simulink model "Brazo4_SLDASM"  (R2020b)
settings: Solver=VariableStepAuto  StartTime=0.0  StopTime=20  RelTol=1e-3
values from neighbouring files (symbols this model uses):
  q = [q 0]    [robotSimulation.m]    (also in robotSimulationWithConstraints.m = [q' 0])
undefined symbols (not defined in the file or in its folder): deg, kg, m, N, rad, s, X, Y, Z
libraries: sm_lib x118, nesl_utility x17, pid_lib x4
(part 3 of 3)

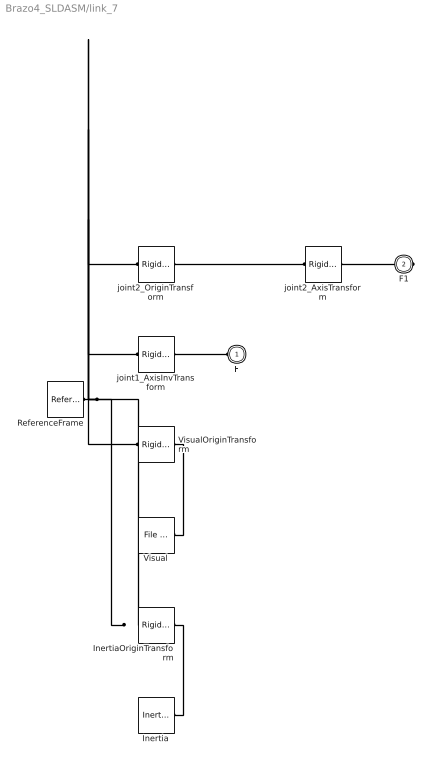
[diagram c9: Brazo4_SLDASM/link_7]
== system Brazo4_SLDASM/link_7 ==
  Inertia : sm_lib/Body Elements/Inertia  InertiaType=Custom  Mass=34.189  MassUnits=kg  CenterOfMass=[0, 0, 0]  CenterOfMassUnits=m  MomentsOfInertia=[0.101, 0.32346, 0.28584]  MomentsOfInertiaUnits=kg*m^2  ProductsOfInertia=[-2.191e-18, 8.7345e-17, 3.6996e-17]  ProductsOfInertiaUnits=kg*m^2  GraphicType=None  MarkerShape=Inertia  MarkerSize=20  GraphicVisPropType=SimpleVisualProperties  GraphicDiffuseColor=[0.5 0.5 0.5]  GraphicSpecularColor=[0.5 0.5 0.5 1.0]  GraphicAmbientColor=[0.15 0.15 0.15 1.0]  GraphicEmissiveColor=[0.0 0.0 0.0 1.0]  GraphicShininess=75  GraphicOpacity=1.0
  InertiaOriginTransform : sm_lib/Frames and Transforms/Rigid Transform  TranslationMethod=Cartesian  TranslationStandardOffset=0  TranslationLengthUnit=m  TranslationStandardAxis=+Z  TranslationCartesianOffset=[0.07391200000000001, 0, -1.2748e-17]  TranslationROffset=0  TranslationROffsetUnits=m  TranslationZOffset=0  TranslationZOffsetUnits=m  TranslationThetaOffset=0  TranslationThetaOffsetUnits=deg  RotationMethod=RotationSequence  RotationAngleUnits=deg  RotationStandardAxis=+Z  RotationAngle=0.0  RotationArbitraryAxis=[0 0 1]  FollAlignAxisA=+X  BaseAlignAxisA=+Y  FollAlignAxisB=+Y  BaseAlignAxisB=+Z  RotationSequenceAxes=BaseAxes  RotationSequence=XYZ  RotationSequenceAngles=[0, 0, 0]  RotationSequenceAnglesUnits=rad  RotationMatrix=[1 0 0; 0 1 0; 0 0 1]
  ReferenceFrame : sm_lib/Frames and Transforms/Reference Frame
  Visual : sm_lib/Body Elements/File Solid  ExtGeomFileName=Brazo4_SLDASM/meshes/link_2.STL  UnitType=Custom  ExtGeomFileUnits=m  StepReaderType=HEX  ExportConvexHullGeometry=off  InertiaType=Custom  Mass=0  MassUnits=kg  CenterOfMass=[0, 0, 0]  CenterOfMassUnits=m  MomentsOfInertia=[0, 0, 0]  MomentsOfInertiaUnits=kg*m^2  ProductsOfInertia=[0, 0, 0]  ProductsOfInertiaUnits=kg*m^2  BasedOnType=DensityFromFile  Density=1000  DensityUnits=kg/m^3  DoExposeReferenceFrame=on  SerializedFrames=<Frames/>  GraphicType=FromGeometry  MarkerShape=Sphere  MarkerSize=10  GraphicVisPropType=SimpleVisualProperties  GraphicDiffuseColor=[0.77647, 0.75686, 0.73725]  GraphicSpecularColor=[0.5 0.5 0.5 1.0]  GraphicAmbientColor=[0.15 0.15 0.15 1.0]  GraphicEmissiveColor=[0.0 0.0 0.0 1.0]  GraphicShininess=75  GraphicOpacity=1
  VisualOriginTransform : sm_lib/Frames and Transforms/Rigid Transform  TranslationMethod=Cartesian  TranslationStandardOffset=0  TranslationLengthUnit=m  TranslationStandardAxis=+Z  TranslationCartesianOffset=[0, 0, 0]  TranslationROffset=0  TranslationROffsetUnits=m  TranslationZOffset=0  TranslationZOffsetUnits=m  TranslationThetaOffset=0  TranslationThetaOffsetUnits=deg  RotationMethod=RotationSequence  RotationAngleUnits=deg  RotationStandardAxis=+Z  RotationAngle=0.0  RotationArbitraryAxis=[0 0 1]  FollAlignAxisA=+X  BaseAlignAxisA=+Y  FollAlignAxisB=+Y  BaseAlignAxisB=+Z  RotationSequenceAxes=BaseAxes  RotationSequence=XYZ  RotationSequenceAngles=[0, 0, 0]  RotationSequenceAnglesUnits=rad  RotationMatrix=[1 0 0; 0 1 0; 0 0 1]
  joint1_AxisInvTransform : sm_lib/Frames and Transforms/Rigid Transform  TranslationMethod=Cartesian  TranslationStandardOffset=0  TranslationLengthUnit=m  TranslationStandardAxis=+Z  TranslationCartesianOffset=[0, 0, 0]  TranslationROffset=0  TranslationROffsetUnits=m  TranslationZOffset=0  TranslationZOffsetUnits=m  TranslationThetaOffset=0  TranslationThetaOffsetUnits=deg  RotationMethod=ArbitraryAxis  RotationAngleUnits=rad  RotationStandardAxis=+Z  RotationAngle=0  RotationArbitraryAxis=[1, 0, 0]  FollAlignAxisA=+X  BaseAlignAxisA=+Y  FollAlignAxisB=+Y  BaseAlignAxisB=+Z  RotationSequenceAxes=FollowerAxes  RotationSequence=XYX  RotationSequenceAngles=[0 0 0]  RotationSequenceAnglesUnits=deg  RotationMatrix=[1 0 0; 0 1 0; 0 0 1]
  joint2_AxisTransform : sm_lib/Frames and Transforms/Rigid Transform  TranslationMethod=Cartesian  TranslationStandardOffset=0  TranslationLengthUnit=m  TranslationStandardAxis=+Z  TranslationCartesianOffset=[0, 0, 0]  TranslationROffset=0  TranslationROffsetUnits=m  TranslationZOffset=0  TranslationZOffsetUnits=m  TranslationThetaOffset=0  TranslationThetaOffsetUnits=deg  RotationMethod=ArbitraryAxis  RotationAngleUnits=rad  RotationStandardAxis=+Z  RotationAngle=0  RotationArbitraryAxis=[1, 0, 0]  FollAlignAxisA=+X  BaseAlignAxisA=+Y  FollAlignAxisB=+Y  BaseAlignAxisB=+Z  RotationSequenceAxes=FollowerAxes  RotationSequence=XYX  RotationSequenceAngles=[0 0 0]  RotationSequenceAnglesUnits=deg  RotationMatrix=[1 0 0; 0 1 0; 0 0 1]
  joint2_OriginTransform : sm_lib/Frames and Transforms/Rigid Transform  TranslationMethod=Cartesian  TranslationStandardOffset=0  TranslationLengthUnit=m  TranslationStandardAxis=+Z  TranslationCartesianOffset=[0.25, 0, 0]  TranslationROffset=0  TranslationROffsetUnits=m  TranslationZOffset=0  TranslationZOffsetUnits=m  TranslationThetaOffset=0  TranslationThetaOffsetUnits=deg  RotationMethod=RotationSequence  RotationAngleUnits=deg  RotationStandardAxis=+Z  RotationAngle=0.0  RotationArbitraryAxis=[0 0 1]  FollAlignAxisA=+X  BaseAlignAxisA=+Y  FollAlignAxisB=+Y  BaseAlignAxisB=+Z  RotationSequenceAxes=BaseAxes  RotationSequence=XYZ  RotationSequenceAngles=[0, 0, 0]  RotationSequenceAnglesUnits=rad  RotationMatrix=[1 0 0; 0 1 0; 0 0 1]
  F : PMIOPort  Side=Left
  F1 : PMIOPort  Port=2  Side=Right
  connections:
  Inertia/RConn1 -- InertiaOriginTransform/RConn1
  ReferenceFrame/RConn1 -- InertiaOriginTransform/LConn1 -- VisualOriginTransform/LConn1 -- joint1_AxisInvTransform/LConn1 -- joint2_OriginTransform/LConn1
  Visual/RConn1 -- VisualOriginTransform/RConn1
  joint1_AxisInvTransform/RConn1 -- F/RConn1
  joint2_AxisTransform/RConn1 -- F1/RConn1
  joint2_AxisTransform/LConn1 -- joint2_OriginTransform/RConn1

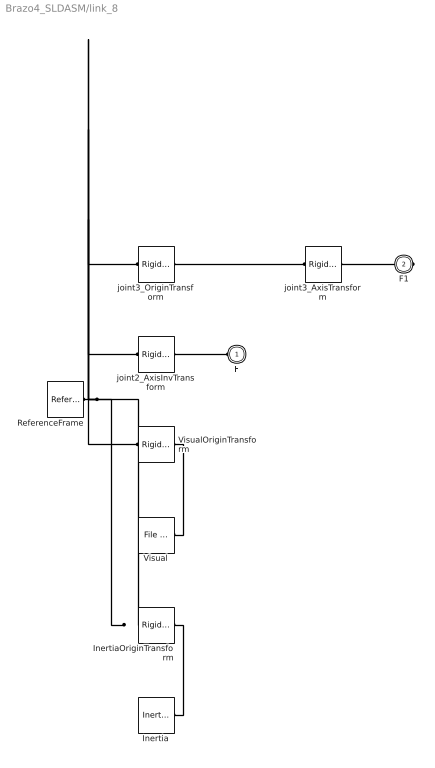
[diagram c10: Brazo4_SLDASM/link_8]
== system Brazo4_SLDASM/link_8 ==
  Inertia : sm_lib/Body Elements/Inertia  InertiaType=Custom  Mass=13.946  MassUnits=kg  CenterOfMass=[0, 0, 0]  CenterOfMassUnits=m  MomentsOfInertia=[0.026465, 0.06281399999999999, 0.054336]  MomentsOfInertiaUnits=kg*m^2  ProductsOfInertia=[-5.1463e-19, 1.9268e-17, 6.4193e-18]  ProductsOfInertiaUnits=kg*m^2  GraphicType=None  MarkerShape=Inertia  MarkerSize=20  GraphicVisPropType=SimpleVisualProperties  GraphicDiffuseColor=[0.5 0.5 0.5]  GraphicSpecularColor=[0.5 0.5 0.5 1.0]  GraphicAmbientColor=[0.15 0.15 0.15 1.0]  GraphicEmissiveColor=[0.0 0.0 0.0 1.0]  GraphicShininess=75  GraphicOpacity=1.0
  InertiaOriginTransform : sm_lib/Frames and Transforms/Rigid Transform  TranslationMethod=Cartesian  TranslationStandardOffset=0  TranslationLengthUnit=m  TranslationStandardAxis=+Z  TranslationCartesianOffset=[0.053841, 0, -3.1131e-17]  TranslationROffset=0  TranslationROffsetUnits=m  TranslationZOffset=0  TranslationZOffsetUnits=m  TranslationThetaOffset=0  TranslationThetaOffsetUnits=deg  RotationMethod=RotationSequence  RotationAngleUnits=deg  RotationStandardAxis=+Z  RotationAngle=0.0  RotationArbitraryAxis=[0 0 1]  FollAlignAxisA=+X  BaseAlignAxisA=+Y  FollAlignAxisB=+Y  BaseAlignAxisB=+Z  RotationSequenceAxes=BaseAxes  RotationSequence=XYZ  RotationSequenceAngles=[0, 0, 0]  RotationSequenceAnglesUnits=rad  RotationMatrix=[1 0 0; 0 1 0; 0 0 1]
  ReferenceFrame : sm_lib/Frames and Transforms/Reference Frame
  Visual : sm_lib/Body Elements/File Solid  ExtGeomFileName=Brazo4_SLDASM/meshes/link_3.STL  UnitType=Custom  ExtGeomFileUnits=m  StepReaderType=HEX  ExportConvexHullGeometry=off  InertiaType=Custom  Mass=0  MassUnits=kg  CenterOfMass=[0, 0, 0]  CenterOfMassUnits=m  MomentsOfInertia=[0, 0, 0]  MomentsOfInertiaUnits=kg*m^2  ProductsOfInertia=[0, 0, 0]  ProductsOfInertiaUnits=kg*m^2  BasedOnType=DensityFromFile  Density=1000  DensityUnits=kg/m^3  DoExposeReferenceFrame=on  SerializedFrames=<Frames/>  GraphicType=FromGeometry  MarkerShape=Sphere  MarkerSize=10  GraphicVisPropType=SimpleVisualProperties  GraphicDiffuseColor=[0.77647, 0.75686, 0.73725]  GraphicSpecularColor=[0.5 0.5 0.5 1.0]  GraphicAmbientColor=[0.15 0.15 0.15 1.0]  GraphicEmissiveColor=[0.0 0.0 0.0 1.0]  GraphicShininess=75  GraphicOpacity=1
  VisualOriginTransform : sm_lib/Frames and Transforms/Rigid Transform  TranslationMethod=Cartesian  TranslationStandardOffset=0  TranslationLengthUnit=m  TranslationStandardAxis=+Z  TranslationCartesianOffset=[0, 0, 0]  TranslationROffset=0  TranslationROffsetUnits=m  TranslationZOffset=0  TranslationZOffsetUnits=m  TranslationThetaOffset=0  TranslationThetaOffsetUnits=deg  RotationMethod=RotationSequence  RotationAngleUnits=deg  RotationStandardAxis=+Z  RotationAngle=0.0  RotationArbitraryAxis=[0 0 1]  FollAlignAxisA=+X  BaseAlignAxisA=+Y  FollAlignAxisB=+Y  BaseAlignAxisB=+Z  RotationSequenceAxes=BaseAxes  RotationSequence=XYZ  RotationSequenceAngles=[0, 0, 0]  RotationSequenceAnglesUnits=rad  RotationMatrix=[1 0 0; 0 1 0; 0 0 1]
  joint2_AxisInvTransform : sm_lib/Frames and Transforms/Rigid Transform  TranslationMethod=Cartesian  TranslationStandardOffset=0  TranslationLengthUnit=m  TranslationStandardAxis=+Z  TranslationCartesianOffset=[0, 0, 0]  TranslationROffset=0  TranslationROffsetUnits=m  TranslationZOffset=0  TranslationZOffsetUnits=m  TranslationThetaOffset=0  TranslationThetaOffsetUnits=deg  RotationMethod=ArbitraryAxis  RotationAngleUnits=rad  RotationStandardAxis=+Z  RotationAngle=0  RotationArbitraryAxis=[1, 0, 0]  FollAlignAxisA=+X  BaseAlignAxisA=+Y  FollAlignAxisB=+Y  BaseAlignAxisB=+Z  RotationSequenceAxes=FollowerAxes  RotationSequence=XYX  RotationSequenceAngles=[0 0 0]  RotationSequenceAnglesUnits=deg  RotationMatrix=[1 0 0; 0 1 0; 0 0 1]
  joint3_AxisTransform : sm_lib/Frames and Transforms/Rigid Transform  TranslationMethod=Cartesian  TranslationStandardOffset=0  TranslationLengthUnit=m  TranslationStandardAxis=+Z  TranslationCartesianOffset=[0, 0, 0]  TranslationROffset=0  TranslationROffsetUnits=m  TranslationZOffset=0  TranslationZOffsetUnits=m  TranslationThetaOffset=0  TranslationThetaOffsetUnits=deg  RotationMethod=ArbitraryAxis  RotationAngleUnits=rad  RotationStandardAxis=+Z  RotationAngle=0  RotationArbitraryAxis=[1, 0, 0]  FollAlignAxisA=+X  BaseAlignAxisA=+Y  FollAlignAxisB=+Y  BaseAlignAxisB=+Z  RotationSequenceAxes=FollowerAxes  RotationSequence=XYX  RotationSequenceAngles=[0 0 0]  RotationSequenceAnglesUnits=deg  RotationMatrix=[1 0 0; 0 1 0; 0 0 1]
  joint3_OriginTransform : sm_lib/Frames and Transforms/Rigid Transform  TranslationMethod=Cartesian  TranslationStandardOffset=0  TranslationLengthUnit=m  TranslationStandardAxis=+Z  TranslationCartesianOffset=[0.16, 0, 0]  TranslationROffset=0  TranslationROffsetUnits=m  TranslationZOffset=0  TranslationZOffsetUnits=m  TranslationThetaOffset=0  TranslationThetaOffsetUnits=deg  RotationMethod=RotationSequence  RotationAngleUnits=deg  RotationStandardAxis=+Z  RotationAngle=0.0  RotationArbitraryAxis=[0 0 1]  FollAlignAxisA=+X  BaseAlignAxisA=+Y  FollAlignAxisB=+Y  BaseAlignAxisB=+Z  RotationSequenceAxes=BaseAxes  RotationSequence=XYZ  RotationSequenceAngles=[0, 0, 0]  RotationSequenceAnglesUnits=rad  RotationMatrix=[1 0 0; 0 1 0; 0 0 1]
  F : PMIOPort  Side=Left
  F1 : PMIOPort  Port=2  Side=Right
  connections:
  Inertia/RConn1 -- InertiaOriginTransform/RConn1
  ReferenceFrame/RConn1 -- InertiaOriginTransform/LConn1 -- VisualOriginTransform/LConn1 -- joint2_AxisInvTransform/LConn1 -- joint3_OriginTransform/LConn1
  Visual/RConn1 -- VisualOriginTransform/RConn1
  joint2_AxisInvTransform/RConn1 -- F/RConn1
  joint3_AxisTransform/RConn1 -- F1/RConn1
  joint3_AxisTransform/LConn1 -- joint3_OriginTransform/RConn1

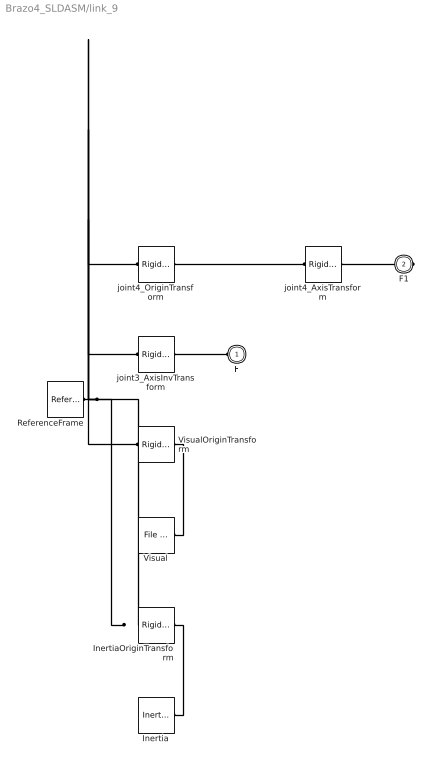
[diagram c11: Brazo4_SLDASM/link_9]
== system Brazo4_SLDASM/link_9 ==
  Inertia : sm_lib/Body Elements/Inertia  InertiaType=Custom  Mass=2.6258  MassUnits=kg  CenterOfMass=[0, 0, 0]  CenterOfMassUnits=m  MomentsOfInertia=[0.0019708, 0.0032587, 0.0021473]  MomentsOfInertiaUnits=kg*m^2  ProductsOfInertia=[-1.2627e-19, -3.1081e-19, 2.4201e-20]  ProductsOfInertiaUnits=kg*m^2  GraphicType=None  MarkerShape=Inertia  MarkerSize=20  GraphicVisPropType=SimpleVisualProperties  GraphicDiffuseColor=[0.5 0.5 0.5]  GraphicSpecularColor=[0.5 0.5 0.5 1.0]  GraphicAmbientColor=[0.15 0.15 0.15 1.0]  GraphicEmissiveColor=[0.0 0.0 0.0 1.0]  GraphicShininess=75  GraphicOpacity=1.0
  InertiaOriginTransform : sm_lib/Frames and Transforms/Rigid Transform  TranslationMethod=Cartesian  TranslationStandardOffset=0  TranslationLengthUnit=m  TranslationStandardAxis=+Z  TranslationCartesianOffset=[0.026026, -5.5511e-17, 3.1752e-17]  TranslationROffset=0  TranslationROffsetUnits=m  TranslationZOffset=0  TranslationZOffsetUnits=m  TranslationThetaOffset=0  TranslationThetaOffsetUnits=deg  RotationMethod=RotationSequence  RotationAngleUnits=deg  RotationStandardAxis=+Z  RotationAngle=0.0  RotationArbitraryAxis=[0 0 1]  FollAlignAxisA=+X  BaseAlignAxisA=+Y  FollAlignAxisB=+Y  BaseAlignAxisB=+Z  RotationSequenceAxes=BaseAxes  RotationSequence=XYZ  RotationSequenceAngles=[0, 0, 0]  RotationSequenceAnglesUnits=rad  RotationMatrix=[1 0 0; 0 1 0; 0 0 1]
  ReferenceFrame : sm_lib/Frames and Transforms/Reference Frame
  Visual : sm_lib/Body Elements/File Solid  ExtGeomFileName=Brazo4_SLDASM/meshes/link_4.STL  UnitType=Custom  ExtGeomFileUnits=m  StepReaderType=HEX  ExportConvexHullGeometry=off  InertiaType=Custom  Mass=0  MassUnits=kg  CenterOfMass=[0, 0, 0]  CenterOfMassUnits=m  MomentsOfInertia=[0, 0, 0]  MomentsOfInertiaUnits=kg*m^2  ProductsOfInertia=[0, 0, 0]  ProductsOfInertiaUnits=kg*m^2  BasedOnType=DensityFromFile  Density=1000  DensityUnits=kg/m^3  DoExposeReferenceFrame=on  SerializedFrames=<Frames/>  GraphicType=FromGeometry  MarkerShape=Sphere  MarkerSize=10  GraphicVisPropType=SimpleVisualProperties  GraphicDiffuseColor=[0.77647, 0.75686, 0.73725]  GraphicSpecularColor=[0.5 0.5 0.5 1.0]  GraphicAmbientColor=[0.15 0.15 0.15 1.0]  GraphicEmissiveColor=[0.0 0.0 0.0 1.0]  GraphicShininess=75  GraphicOpacity=1
  VisualOriginTransform : sm_lib/Frames and Transforms/Rigid Transform  TranslationMethod=Cartesian  TranslationStandardOffset=0  TranslationLengthUnit=m  TranslationStandardAxis=+Z  TranslationCartesianOffset=[0, 0, 0]  TranslationROffset=0  TranslationROffsetUnits=m  TranslationZOffset=0  TranslationZOffsetUnits=m  TranslationThetaOffset=0  TranslationThetaOffsetUnits=deg  RotationMethod=RotationSequence  RotationAngleUnits=deg  RotationStandardAxis=+Z  RotationAngle=0.0  RotationArbitraryAxis=[0 0 1]  FollAlignAxisA=+X  BaseAlignAxisA=+Y  FollAlignAxisB=+Y  BaseAlignAxisB=+Z  RotationSequenceAxes=BaseAxes  RotationSequence=XYZ  RotationSequenceAngles=[0, 0, 0]  RotationSequenceAnglesUnits=rad  RotationMatrix=[1 0 0; 0 1 0; 0 0 1]
  joint3_AxisInvTransform : sm_lib/Frames and Transforms/Rigid Transform  TranslationMethod=Cartesian  TranslationStandardOffset=0  TranslationLengthUnit=m  TranslationStandardAxis=+Z  TranslationCartesianOffset=[0, 0, 0]  TranslationROffset=0  TranslationROffsetUnits=m  TranslationZOffset=0  TranslationZOffsetUnits=m  TranslationThetaOffset=0  TranslationThetaOffsetUnits=deg  RotationMethod=ArbitraryAxis  RotationAngleUnits=rad  RotationStandardAxis=+Z  RotationAngle=0  RotationArbitraryAxis=[1, 0, 0]  FollAlignAxisA=+X  BaseAlignAxisA=+Y  FollAlignAxisB=+Y  BaseAlignAxisB=+Z  RotationSequenceAxes=FollowerAxes  RotationSequence=XYX  RotationSequenceAngles=[0 0 0]  RotationSequenceAnglesUnits=deg  RotationMatrix=[1 0 0; 0 1 0; 0 0 1]
  joint4_AxisTransform : sm_lib/Frames and Transforms/Rigid Transform  TranslationMethod=Cartesian  TranslationStandardOffset=0  TranslationLengthUnit=m  TranslationStandardAxis=+Z  TranslationCartesianOffset=[0, 0, 0]  TranslationROffset=0  TranslationROffsetUnits=m  TranslationZOffset=0  TranslationZOffsetUnits=m  TranslationThetaOffset=0  TranslationThetaOffsetUnits=deg  RotationMethod=ArbitraryAxis  RotationAngleUnits=rad  RotationStandardAxis=+Z  RotationAngle=0  RotationArbitraryAxis=[1, 0, 0]  FollAlignAxisA=+X  BaseAlignAxisA=+Y  FollAlignAxisB=+Y  BaseAlignAxisB=+Z  RotationSequenceAxes=FollowerAxes  RotationSequence=XYX  RotationSequenceAngles=[0 0 0]  RotationSequenceAnglesUnits=deg  RotationMatrix=[1 0 0; 0 1 0; 0 0 1]
  joint4_OriginTransform : sm_lib/Frames and Transforms/Rigid Transform  TranslationMethod=Cartesian  TranslationStandardOffset=0  TranslationLengthUnit=m  TranslationStandardAxis=+Z  TranslationCartesianOffset=[0, 0, 0]  TranslationROffset=0  TranslationROffsetUnits=m  TranslationZOffset=0  TranslationZOffsetUnits=m  TranslationThetaOffset=0  TranslationThetaOffsetUnits=deg  RotationMethod=RotationSequence  RotationAngleUnits=deg  RotationStandardAxis=+Z  RotationAngle=0.0  RotationArbitraryAxis=[0 0 1]  FollAlignAxisA=+X  BaseAlignAxisA=+Y  FollAlignAxisB=+Y  BaseAlignAxisB=+Z  RotationSequenceAxes=BaseAxes  RotationSequence=XYZ  RotationSequenceAngles=[1.5708, 0, 1.5708]  RotationSequenceAnglesUnits=rad  RotationMatrix=[1 0 0; 0 1 0; 0 0 1]
  F : PMIOPort  Side=Left
  F1 : PMIOPort  Port=2  Side=Right
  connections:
  Inertia/RConn1 -- InertiaOriginTransform/RConn1
  ReferenceFrame/RConn1 -- InertiaOriginTransform/LConn1 -- VisualOriginTransform/LConn1 -- joint3_AxisInvTransform/LConn1 -- joint4_OriginTransform/LConn1
  Visual/RConn1 -- VisualOriginTransform/RConn1
  joint3_AxisInvTransform/RConn1 -- F/RConn1
  joint4_AxisTransform/RConn1 -- F1/RConn1
  joint4_AxisTransform/LConn1 -- joint4_OriginTransform/RConn1
